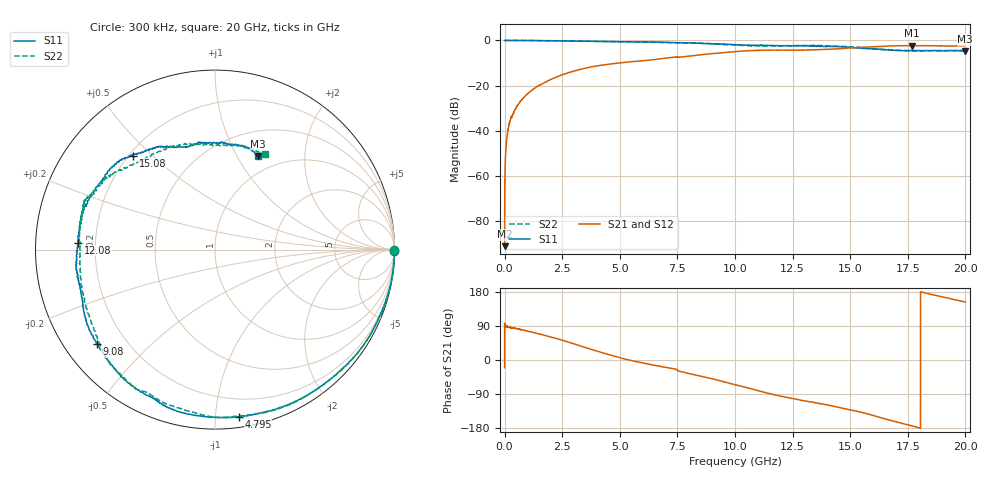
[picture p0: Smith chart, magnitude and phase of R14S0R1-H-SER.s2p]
!{R14S0R1}
!Johanson Technology Inc.
!www.johansontechnology.com
!Test Board Conditions:
!Substrate Type  RO4350B
!Substrate Thickness  20 mil
!Substrate Dk  3.66
!TL Type: GCPW
!TL Trace Width  36 mil
!TL Gap  12 mil
!Electrode orientation  Horizontal
!DUT TOPOLOGY	SERIES
!Mounting Pad LxW  26x36 mil
! Created Wed Nov 25 17:33:21 2020
! 2 Port Network Data from SP1.SP block
! freq  magS11  angS11  magS21  angS21  magS12  angS12  magS22  angS22
# khz S ma R 50
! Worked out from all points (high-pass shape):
!   20001 points, 300 kHz to 20 GHz, reference 50 ohm
!   highest |S21| = -2.28 dB at 17.66 GHz (marker M1); lowest = -91.0 dB at 300 kHz (marker M2)
!   |S21| within 3 dB of the highest: 9.603234 GHz to 9.603392 GHz (158 kHz wide, 0.00164 % of centre); 9.614 GHz to end of sweep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
!   lowest |S11| = -4.8 dB at 20 GHz (marker M3), VSWR 3.70, Z = 39.4 + j61.5 ohm
!   |S11| at or under -10 dB: nowhere
!   |S22| runs from -4.8 to 0.0 dB; largest |S21 - S12| = 0.021
!   S11 on the Smith chart (normalised r, x): 300 kHz: open; 4.795 GHz: 0.07, -1.15; 9.08 GHz: 0.10, -0.35; 12.08 GHz: 0.13, +0.03; 15.08 GHz: 0.22, +0.44; 20 GHz: 0.79, +1.23
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300  0.9967 -0.5  2.825e-05 -20.3  0.0001103 118.3  0.9985 -0.3
105300  1 -1.5  0.007481 88.6  0.007469 88.0  0.9992 -1.5
156300  0.9999 -2.3  0.01106 87.3  0.01108 87.3  0.9981 -2.3
292300  0.999 -4.2  0.02072 85.2  0.02079 85.3  0.9996 -4.3
563300  0.9992 -7.5  0.03661 82.2  0.03676 82.1  0.9988 -7.5
1399300  0.9914 -19.7  0.09509 70.2  0.09541 70.1  0.9927 -19.8
2357300  0.9819 -34.9  0.1636 54.7  0.1639 54.6  0.9824 -35.4
3334300  0.9626 -53.4  0.2327 36.2  0.2332 36.2  0.9632 -53.9
4795300  0.9406 -81.9  0.3102 9.4  0.3111 9.6  0.9394 -78.9
5771300  0.9288 -97.8  0.3487 -5.0  0.3496 -5.0  0.9314 -91.7
6667300  0.916 -107.3  0.388 -15.8  0.3889 -15.5  0.9058 -103.1
7600300  0.8943 -117.6  0.4283 -29.9  0.432 -29.8  0.889 -120.8
9080300  0.843 -141.5  0.515 -50.6  0.5182 -51.0  0.8419 -138.6
1.00003e7  0.8069 -155.2  0.5667 -65.2  0.57 -65.1  0.7921 -153.7
1.20793e7  0.7631 177.0  0.6122 -96.5  0.6111 -97.0  0.7678 169.3
1.33343e7  0.7522 156.9  0.6211 -111.2  0.6166 -111.6  0.7722 160.7
1.50753e7  0.6949 131.1  0.6845 -132.5  0.6803 -132.3  0.7221 145.4
1.66673e7  0.6156 112.2  0.7515 -157.9  0.7525 -156.5  0.629 114.8
1.76643e7  0.5978 99.1  0.769 -173.7  0.7726 -173.6  0.5851 93.2
1.88233e7  0.592 83.4  0.7614 168.9  0.7605 168.8  0.5934 72.0
1.99953e7  0.5749 65.3  0.7653 153.2  0.7665 154.0  0.6011 62.5
2e7  0.5759 65.3  0.7678 153.2  0.7672 154.0  0.6005 62.6
